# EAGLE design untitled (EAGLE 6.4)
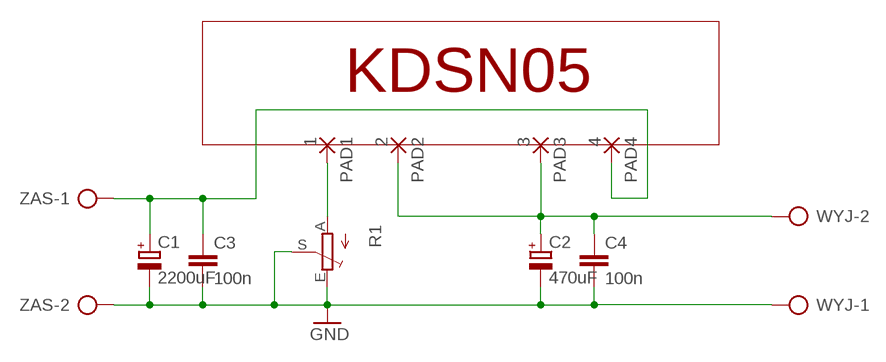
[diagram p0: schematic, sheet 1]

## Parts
C1  2200uF  CPOL-EUE7.5-18  [E7,5-18]
C2  470uF  CPOL-EUE3.5-8  [E3,5-8]
C3  100n  C-EU025-025X050  [C025-025X050]
C4  100n  C-EU025-025X050  [C025-025X050]
PAD1  1  WIREPAD4,16O1,6  [4,16O1,6]
PAD2  2  WIREPAD4,16O1,6  [4,16O1,6]
PAD3  3  WIREPAD4,16O1,6  [4,16O1,6]
PAD4  4  WIREPAD4,16O1,6  [4,16O1,6]
R1  TRIM_EU-S43P  [SP19L]
WYJ  AK300/2  [AK300/2]
ZAS  AK300/2  [AK300/2]

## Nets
GND: C1.- C2.- C3.2 C4.2 R1.E R1.S WYJ.1 ZAS.2
N$1: PAD1.1(P) R1.A
N$3: C1.+ C3.1 PAD4.1(P) ZAS.1
N$4: C2.+ C4.1 PAD2.1(P) PAD3.1(P) WYJ.2

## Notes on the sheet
- KDSN05

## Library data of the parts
C1 C2 = rcl:CPOL-EU: POLARIZED CAPACITOR, European symbol
C3 C4 = rcl:C-EU: CAPACITOR, European symbol
PAD1-PAD4 = wirepad:WIREPAD: Wire PAD connect wire on PCB
R1 = pot:TRIM_EU-: POTENTIOMETER
WYJ ZAS = con-ptr500:AK300/2: CONNECTOR; OC_FARNELL: unknown; OC_NEWARK: unknown

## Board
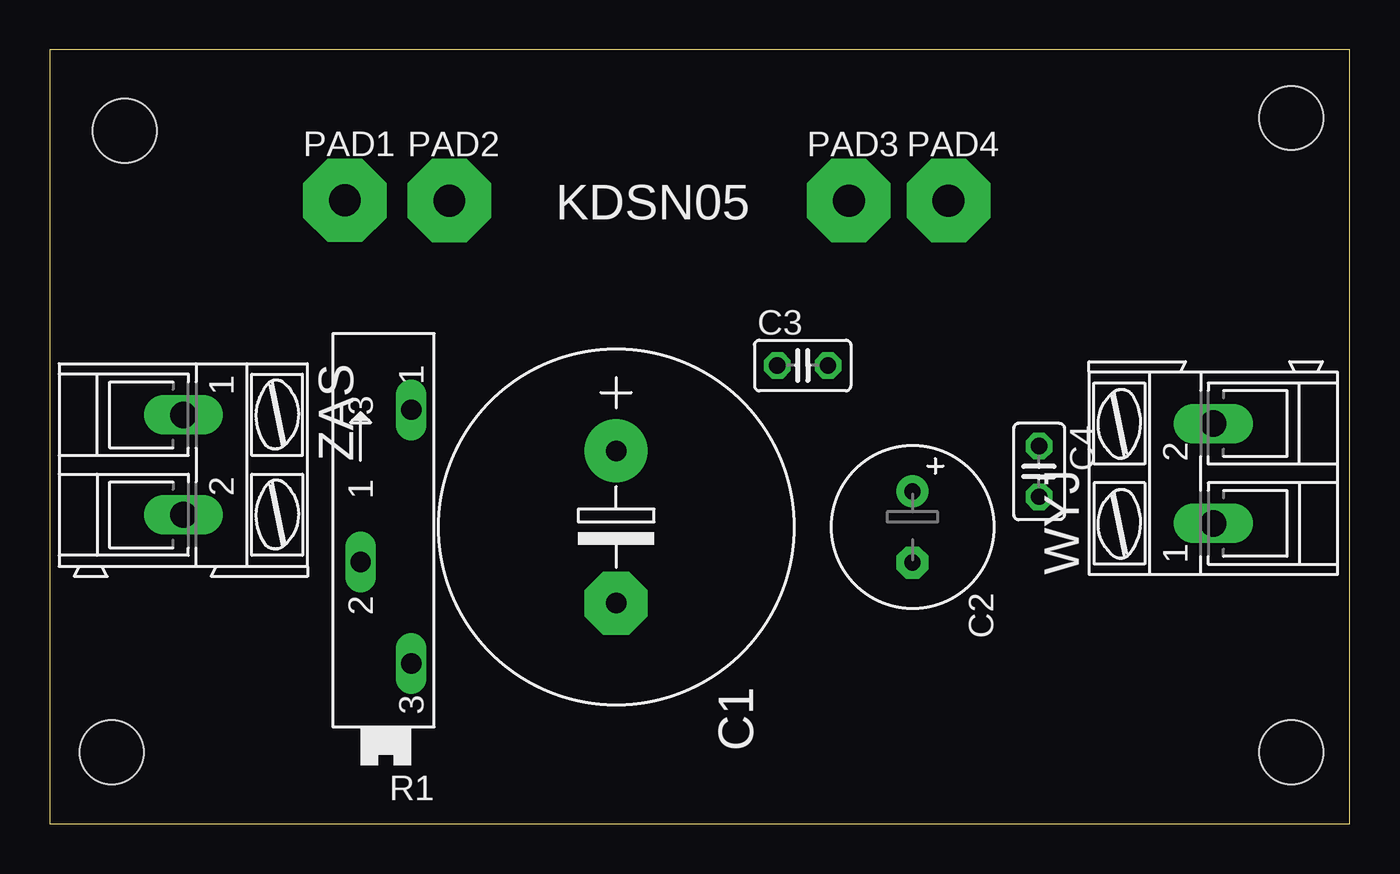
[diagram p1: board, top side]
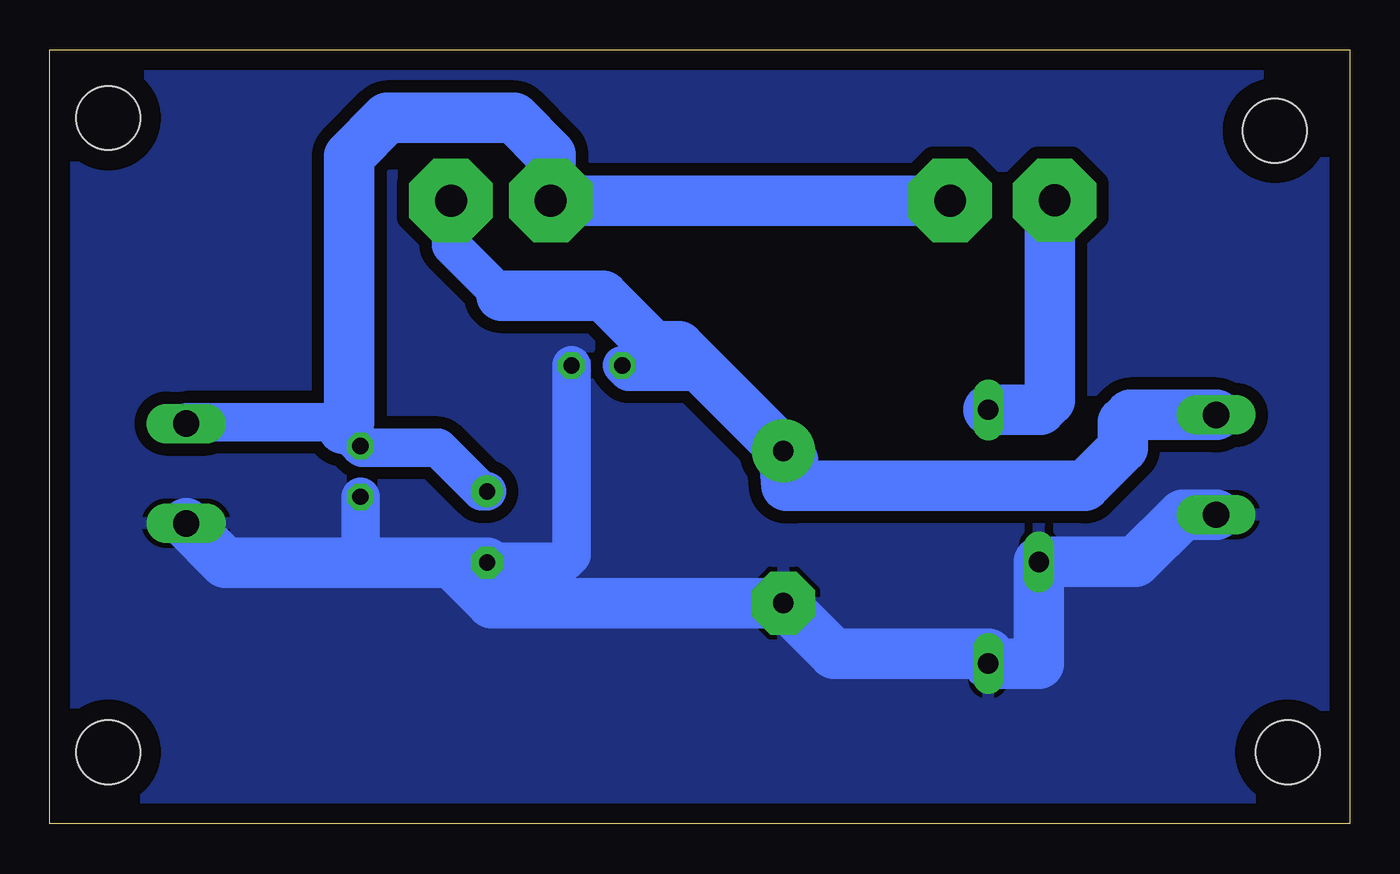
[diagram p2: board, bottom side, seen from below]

Size 65.08 x 38.73 mm. Coordinates in mm from the lower left corner, seen from the top.
Outline: 0,0 65.08,0 65.08,38.73 0,38.73 0,0
Copper layers (1*16): Top 0.035mm / dielectric 1.5mm / Bottom 0.035mm
Design rules "default": minimum track width 10mil, minimum drill 24mil, track to track 8mil, track to pad 8mil, pad to pad 8mil, via to via 8mil, smd to smd 8mil, copper to edge 40mil, drill to drill 8mil, minimum pad ring 10mil, minimum via ring 8mil, stop-mask expansion 4mil, vias tented up to drill 0mil, thermal gap 10mil
Holes 3.2 mm at 3.73,34.69 62.16,35.33 3.1,3.57 62.16,3.57

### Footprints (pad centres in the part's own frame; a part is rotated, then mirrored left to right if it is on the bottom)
E7,5-18 = drill 1.016 pad 3.15: + -3.81,0 | drill 1.016 pad 3.15 octagon: - 3.81,0
E3,5-8 = drill 0.813 pad 1.6: + -1.778,0 | drill 0.813 pad 1.6 octagon: - 1.778,0
C025-025X050 = drill 0.813 octagon: 1 -1.27,0; 2 1.27,0
4,16O1,6 = drill 1.6 pad 4.166 octagon: 1 0,0
SP19L = drill 1.016 long: A 5.715,-1.27; E -6.985,-1.27; S -1.905,1.27
AK300/2 = drill 1.321 long: 1 -2.515,0; 2 2.489,0

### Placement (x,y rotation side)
C1  28.35,14.85 270 top
C2  43.19,14.85 270 top
C3  37.69,22.93 0 top
C4  49.53,17.63 270 top
PAD1  14.77,31.2 0 top
PAD2  20,31.19 0 top
PAD3  40,31.19 0 top
PAD4  45,31.19 0 top
R1  16.83,15 90 top
WYJ  58.25,17.54 90 top
ZAS  6.68,17.95 270 top

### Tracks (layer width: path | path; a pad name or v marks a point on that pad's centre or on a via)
GND
  Bottom 1.93: C4.2 49.53,13.54 50,13.07 | C3.2 38.97,13.43 39.3,13.1 43.71,13.1 43.74,13.07
  Bottom 2.54: ZAS.2 8.36,15.46 10.72,13.1 R1.S 15.55,8.02 R1.E 18.09,8.5 25.81,8.5 C1.- 42.97,11.04 45,13.07 | C2.- 43.74,13.07 45,13.07 | 45,13.07 50,13.07 56.3,13.07 WYJ.1
  pour Bottom (isolate 0.61): 0,36.19 -0.08,36.19 -0.08,38.5 65.33,38.5 65.33,-0.23 -0.08,-0.23 -0.08,35.96 0,35.96
N$1
  Bottom 2.54: R1.A 15.48,20.71 15,21.19 15,30.97 PAD1.1
N$3
  Bottom 1.93: C1.+ 32.31,22.63 36.11,22.63 C3.1 | PAD4.1 45,28.96 42.47,26.43
  Bottom 2.54: ZAS.1 10.98,20.46 11.35,20.09 11.35,18.82 13.26,16.91 27.87,16.91 | 27.87,16.91 28.2,16.91 C1.+ | 42.47,26.43 37.39,26.43 34.85,23.89 33.58,23.89 27.87,18.18 27.87,16.91
N$4
  Bottom 1.93: C2.+ 43.46,16.63 45.64,18.82 49.44,18.82 C4.1 50.41,19.77 50.72,20.09 58.2,20.09 WYJ.2
  Bottom 2.54: 19.61,30.8 PAD2.1 PAD3.1 40,33.49 41.83,35.33 48.19,35.33 50.09,33.42 50.09,20.09 50.41,19.77

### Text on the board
tNames: KDSN05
